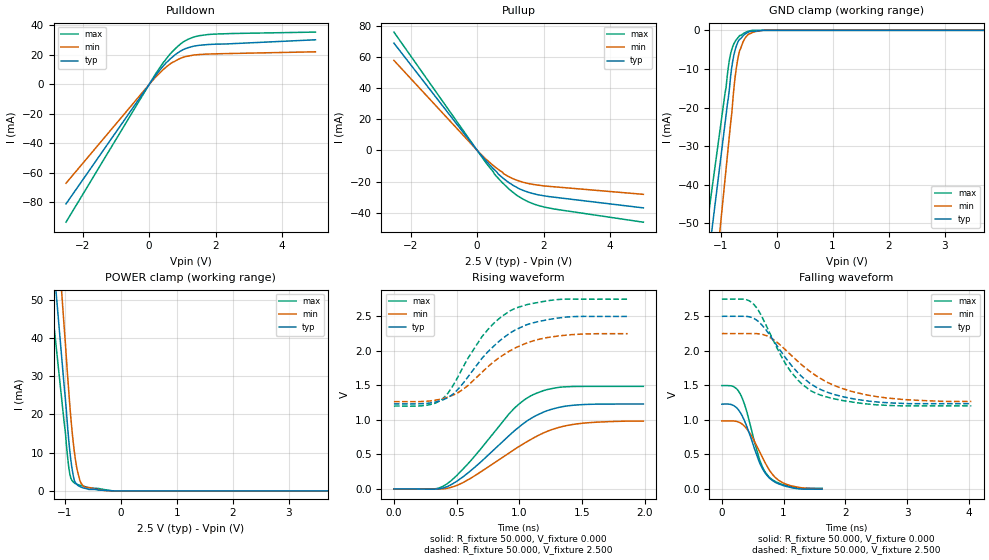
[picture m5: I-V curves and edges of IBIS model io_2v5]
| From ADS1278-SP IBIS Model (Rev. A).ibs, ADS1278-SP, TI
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[Model]   io_2v5
Model_type I/O
Vinl=7.500E-01
Vinh=1.750E+00
Vref=0.000E+00
Rref=1.000E+06
Cref=2.000E-11
Vmeas=1.250E+00
C_comp   698.00E-15   698.00E-15   698.00E-15
[Voltage Range]   2.500E+00   2.250E+00   2.750E+00
[POWER Clamp Reference]   2.500E+00   2.250E+00   2.750E+00
[GND Clamp Reference]   0.000E+00   0.000E+00   0.000E+00
[Pullup Reference]   2.500E+00   2.250E+00   2.750E+00
[Pulldown Reference]   0.000E+00   0.000E+00   0.000E+00
[Temperature Range]   25   105   -40
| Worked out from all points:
|   slope of the pulldown table from 0 to 0.375 V, typ, clamps not added: 33.5 ohm
|   slope of the pullup table from 0 to 0.375 V, typ, clamps not added: 40.7 ohm
|   GND clamp passes 1 mA (typ) near -0.57 V on its own axis
|   POWER clamp passes 1 mA (typ) near -0.71 V on its own axis
|   rising waveform, R_fixture 50.000, V_fixture 0.000: 20-80 % time 462ps typ, 515ps min, 416ps max; typ from 0 V to 1.23 V
|   falling waveform, R_fixture 50.000, V_fixture 0.000: 20-80 % time 323ps typ, 365ps min, 287ps max; typ from 1.23 V to -0.007 V
|   rising waveform, R_fixture 50.000, V_fixture 2.500: 20-80 % time 385ps typ, 415ps min, 345ps max; typ from 1.23 V to 2.5 V
|   falling waveform, R_fixture 50.000, V_fixture 2.500: 20-80 % time 741ps typ, 938ps min, 628ps max; typ from 2.5 V to 1.23 V
[GND Clamp]
-2.5V     -210.5mA   -268.7mA   -184.7mA
-2.46V    -205.4mA   -262.9mA   -180.4mA
-920mV    -24.11mA   -38.58mA   -16.25mA
-900mV    -21.78mA   -35.67mA   -14.61mA
-860mV    -17.37mA   -29.84mA   -9.408mA
-820mV    -11.83mA   -24.02mA   -6.071mA
-780mV    -7.742mA   -17.95mA   -4.085mA
-720mV    -4.13mA    -9.941mA   -2.446mA
-660mV    -2.382mA   -5.288mA   -1.337mA
-520mV    -602uA     -1.268mA   -295.4uA
-220mV    0A         0A         0A
5V        0A         0A         0A
[Power Clamp]
-2.51V    283mA      349.9mA    226.6mA
-2.47V    275.7mA    341.7mA    221.1mA
-1.01V    27.43mA    42.88mA    17.87mA
-930mV    13.52mA    26.46mA    6.392mA
-910mV    10.49mA    22.56mA    4.518mA
-870mV    5.927mA    15.84mA    2.728mA
-830mV    2.78mA     10.44mA    2.119mA
-810mV    2.165mA    8.267mA    1.894mA
-730mV    1.147mA    2.759mA    1.465mA
-630mV    650.3uA    890.9uA    1.091mA
-270mV    149.8uA    48.29uA    297.1uA
5.01V     0A         0A         0A
[Pullup]
-2.51V    68.88mA    57.79mA    75.96mA
30mV      -788.7uA   -677.4uA   -921.9uA
250mV     -6.282mA   -5.354mA   -7.496mA
550mV     -13.02mA   -10.85mA   -15.92mA
630mV     -15.1mA    -12.15mA   -17.78mA
770mV     -17.66mA   -14.15mA   -20.95mA
790mV     -18.03mA   -14.9mA    -21.38mA
1.19V     -23.73mA   -19.12mA   -28.8mA
1.55V     -26.93mA   -21.31mA   -33.13mA
2.09V     -29.42mA   -22.98mA   -36.72mA
5.01V     -36.94mA   -28.23mA   -46.12mA
[Pulldown]
-2.5V     -80.96mA   -66.97mA   -93.37mA
200mV     6.311mA    5.118mA    7.386mA
440mV     12.94mA    10.41mA    15.32mA
640mV     17.52mA    14.1mA     20.92mA
960mV     22.86mA    17.9mA     27.8mA
1.18V     24.97mA    19.29mA    30.76mA
1.36V     26.07mA    20mA       32.31mA
1.78V     27.11mA    20.65mA    33.9mA
5V        30.31mA    22.16mA    35.53mA
[Rising Waveform]
R_fixture = 50.000
V_fixture = 0.000
V_fixture_min = 0.000
V_fixture_max = 0.000
|  time   V(typ)   V(min)   V(max)
0s        0V         0V         0V
320ps     -2.995mV   -2.399mV   698.8uV
420ps     30.33mV    7.797mV    69.91mV
605ps     253.1mV    147.1mV    392.6mV
955ps     832.4mV    565.1mV    1.159V
1.05ns    970mV      672.7mV    1.303V
1.145ns   1.073V     769.5mV    1.393V
1.29ns    1.17V      877.4mV    1.465V
1.445ns   1.215V     939.1mV    1.485V
1.99ns    1.231V     983.3mV    1.487V
[Falling Waveform]
R_fixture = 50.000
V_fixture = 0.000
V_fixture_min = 0.000
V_fixture_max = 0.000
|  time   V(typ)   V(min)   V(max)
0s        1.226V     983.3mV    1.495V
200ps     1.201V     981mV      1.476V
300ps     1.104V     953.9mV    1.37V
395ps     924.1mV    878.6mV    1.145V
610ps     380.2mV    540.8mV    425.7mV
680ps     256.8mV    413.3mV    276.1mV
765ps     159.6mV    276.2mV    171mV
890ps     81.31mV    143.7mV    93.93mV
1.055ns   30.76mV    61.17mV    44.61mV
1.625ns   -6.59mV    0V         5.775mV
[Rising Waveform]
R_fixture = 50.000
V_fixture = 2.500
V_fixture_min = 2.250
V_fixture_max = 2.750
|  time   V(typ)   V(min)   V(max)
0s        1.233V     1.265V     1.202V
250ps     1.238V     1.27V      1.21V
385ps     1.286V     1.306V     1.301V
500ps     1.424V     1.384V     1.588V
710ps     1.909V     1.704V     2.224V
835ps     2.133V     1.896V     2.463V
960ps     2.296V     2.036V     2.611V
1.105ns   2.405V     2.143V     2.688V
1.31ns    2.477V     2.217V     2.745V
1.865ns   2.5V       2.25V      2.75V
[Falling Waveform]
R_fixture = 50.000
V_fixture = 2.500
V_fixture_min = 2.250
V_fixture_max = 2.750
|  time   V(typ)   V(min)   V(max)
0s        2.5V       2.25V      2.75V
360ps     2.5V       2.25V      2.748V
515ps     2.471V     2.25V      2.676V
745ps     2.267V     2.211V     2.317V
1.12ns    1.796V     1.938V     1.693V
1.315ns   1.609V     1.781V     1.505V
1.53ns    1.471V     1.636V     1.381V
1.93ns    1.34V      1.459V     1.283V
2.42ns    1.266V     1.348V     1.223V
4.04ns    1.233V     1.265V     1.202V
[Ramp]
dV/dt_r   7.397E-01/4.612E-10   5.902E-01/5.139E-10   8.935E-01/4.161E-10
dV/dt_f   7.602E-01/7.378E-10   5.911E-01/9.380E-10   9.290E-01/6.274E-10
R_load = 50
